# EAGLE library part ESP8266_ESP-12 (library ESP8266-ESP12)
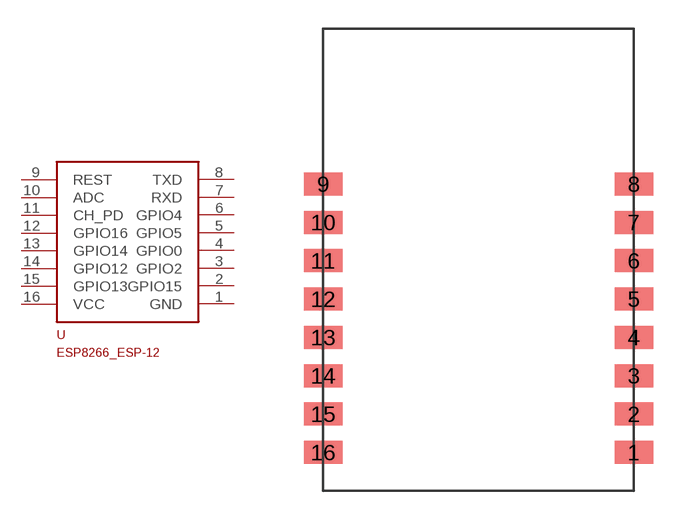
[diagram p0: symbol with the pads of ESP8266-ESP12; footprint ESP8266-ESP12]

Designator prefix -

## ESP8266_ESP-12  [ESP8266-ESP12]
1  GND
2  GPIO15
3  GPIO2
4  GPIO0
5  GPIO5
6  GPIO4
7  RXD
8  TXD
9  REST
10  ADC
11  CH_PD
12  GPIO16
13  GPIO14
14  GPIO12
15  GPIO13
16  VCC

## Footprint ESP8266-ESP12 (pad centres in mm)
smd 2 x 1.2: 1 16.2,2; 2 16.2,4; 3 16.2,6; 4 16.2,8; 5 16.2,10; 6 16.2,12; 7 16.2,14; 8 16.2,16; 9 0,16; 10 0,14; 11 0,12; 12 0,10; 13 0,8; 14 0,6; 15 0,4; 16 0,2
